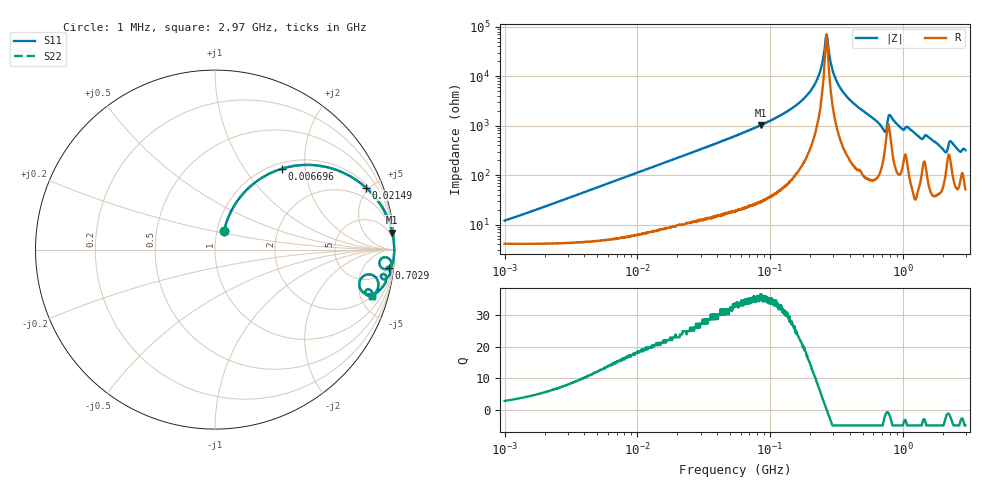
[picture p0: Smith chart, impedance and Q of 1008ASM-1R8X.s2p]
!s-Parameter Generated by FASTRON Sdn. Bhd.
!FASTRON P/N : 1008ASM-1R8X
!Keysight Technologies: E4991B_MY54100416_A.01.15
!Date: Tue Nov 21 10:04:49 2023
!Version  :Rev00  Wed Nov 22 15:07:25 2023
!Data & Calibration Information:
!Freq  S11  S21  S12  S22
!PortZ  Port1:50+j0  Port2:50+j0
!When reading reference impedance value at option line is always used.
! Remarks : This data is being provided solely for informational purposes.
# Hz S dB R 50
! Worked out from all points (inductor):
!   1599 points, 1 MHz to 2.97 GHz, reference 50 ohm
!   read as one part in series: L = 1.81 uH near 1.083 MHz
!   highest Q = 35.8 at 85.93 MHz (marker M1), where L = 1.92 uH
!   self-resonance near 266.3 MHz
!   S11 on the Smith chart (normalised r, x): 1 MHz: 1.08, +0.23; 6.696 MHz: 1.10, +1.51; 21.49 MHz: 1.20, +4.78; 702.9 MHz: 4, -18; 2.97 GHz: 2.03, -6.30
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1000000  -18.80 63.9  -0.40 -6.2  -0.40 -6.2  -18.80 63.9
3804036  -8.34 61.8  -1.06 -22.4  -1.06 -22.4  -8.34 61.8
6696013  -4.67 50.5  -2.24 -35.7  -2.24 -35.7  -4.67 50.5
1.439846e7  -1.60 31.1  -5.73 -56.2  -5.73 -56.2  -1.60 31.1
2.148682e7  -0.83 22.3  -8.39 -65.3  -8.39 -65.3  -0.83 22.3
5.477226e7  -0.15 9.1  -16.00 -79.2  -16.00 -79.2  -0.15 9.1
8.593077e7  -0.06 5.5  -20.40 -82.9  -20.40 -82.9  -0.06 5.5
1.505037e8  -0.02 2.4  -27.50 -85.4  -27.50 -85.4  -0.02 2.4
2.073156e8  -0.01 1.0  -34.90 -84.5  -34.90 -84.5  -0.01 1.0
2.373059e8  -0.01 0.5  -41.50 -80.1  -41.50 -80.1  -0.01 0.5
2.675872e8  -0.01 -0.0  -56.90 7.3  -56.90 7.3  -0.01 -0.0
2.987278e8  -0.01 -0.5  -41.80 79.3  -41.80 79.3  -0.01 -0.5
3.402349e8  -0.01 -1.0  -35.10 83.9  -35.10 83.9  -0.01 -1.0
7.028992e8  -0.22 -6.1  -19.30 73.6  -19.30 73.6  -0.22 -6.1
7.38967e8  -0.61 -6.2  -18.10 54.0  -18.10 54.0  -0.61 -6.2
7.846996e8  -0.36 -2.6  -24.40 46.8  -24.40 46.8  -0.36 -2.6
9.878038e8  -0.20 -6.5  -18.90 75.0  -18.90 75.0  -0.20 -6.5
1.629261e9  -0.28 -10.3  -14.90 74.9  -14.90 74.9  -0.28 -10.3
2.061253e9  -1.01 -16.3  -10.80 59.9  -10.80 59.9  -1.01 -16.3
2.289646e9  -0.82 -9.9  -14.60 56.5  -14.60 56.5  -0.82 -9.9
2.660507e9  -0.88 -16.6  -10.70 62.5  -10.70 62.5  -0.88 -16.6
2.970126e9  -0.79 -16.4  -10.90 64.3  -10.90 64.3  -0.79 -16.4
